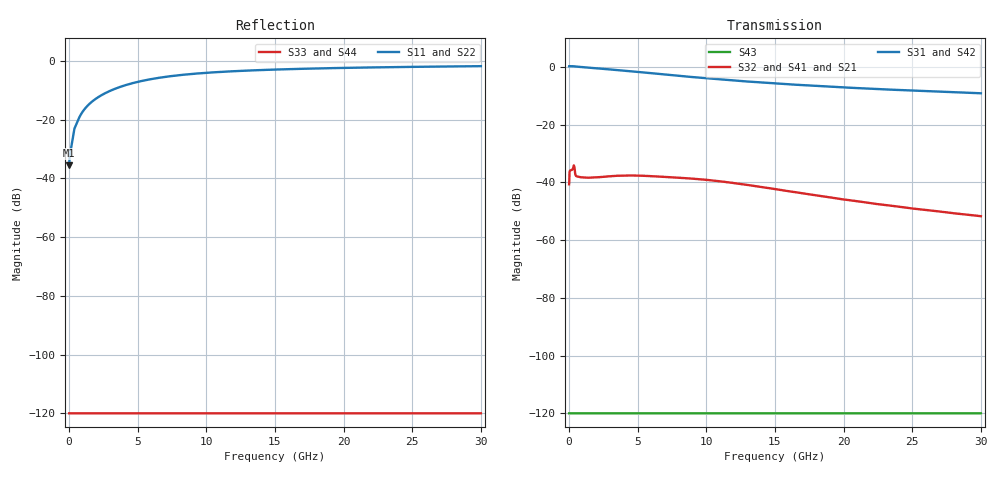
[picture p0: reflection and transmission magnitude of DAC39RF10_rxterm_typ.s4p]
! Copyright 2008, Texas Instruments Incorporated. All rights reserved.
! Generated by program util_convert_RxTerm_to_s4p on 03-29-2011 13:58:47
!  1 ----xxxxxxxxxxxxxxxxxx---- 3
!  xxxxxxxxxxxxxxxxxx
!  (Input) xxxxxxxxxxxxxxxxxx  (Output)
!  xxxxxxxxxxxxxxxxxx
!  2 ----xxxxxxxxxxxxxxxxxx---- 4
! FREQ  S11  S12  S13  S14
!  S21  S22  S23  S24
!  S31  S32  S33  S34
!  S41  S42  S43  S44
!  DB  ANG  DB  ANG  DB  ANG  DB  ANG
# HZ S DB R 50.00
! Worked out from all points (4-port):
!   3000 points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, 10 MHz to 30 GHz, reference 50 ohm
!   strongest paths, dB at 10 MHz, 7.51 GHz, 15.01 GHz, 22.51 GHz, 30 GHz:
!     S31: 0.1, -2.9, -5.8, -7.7, -9.2
!     S42: 0.2, -2.9, -5.8, -7.8, -9.2
!     S32: -40.7, -38.3, -42.4, -47.6, -51.7
!     S41: -40.7, -38.5, -42.4, -47.6, -51.7
!     S21: -40.7, -38.5, -42.4, -47.6, -51.7
!     S43: -120.0, -120.0, -120.0, -120.0, -120.0
!   lowest |S11| = -35.5 dB at 20 MHz (marker M1), VSWR 1.03, Z = 51.7 + j0.154 ohm
!   |S11| at or under -10 dB: start of sweep to 3.086 GHz
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1e7  -35.14 -9.5  -40.70 -7.4  -120.00 0.0  -120.00 0.0
     -40.69 -7.7  -35.04 -9.3  -120.00 0.0  -120.00 0.0
     0.15 -0.2  -40.70 -7.4  -120.00 0.0  -120.00 0.0
     -40.69 -7.7  0.15 -0.2  -120.00 0.0  -120.00 0.0
2e7  -35.53 5.1  -40.08 29.0  -120.00 0.0  -120.00 0.0
     -40.17 28.8  -35.40 5.0  -120.00 0.0  -120.00 0.0
     0.14 0.1  -40.08 29.0  -120.00 0.0  -120.00 0.0
     -40.17 28.8  0.15 0.1  -120.00 0.0  -120.00 0.0
5e8  -21.95 -86.1  -37.78 -19.3  -120.00 0.0  -120.00 0.0
     -37.74 -19.6  -21.88 -86.0  -120.00 0.0  -120.00 0.0
     0.07 -4.5  -37.78 -19.3  -120.00 0.0  -120.00 0.0
     -37.74 -19.6  0.08 -4.6  -120.00 0.0  -120.00 0.0
1.28e9  -15.61 -104.9  -38.41 -11.2  -120.00 0.0  -120.00 0.0
        -38.43 -11.6  -15.54 -105.1  -120.00 0.0  -120.00 0.0
        -0.26 -9.5  -38.41 -11.2  -120.00 0.0  -120.00 0.0
        -38.43 -11.6  -0.26 -9.6  -120.00 0.0  -120.00 0.0
5.1e9  -7.03 -127.4  -37.70 -32.9  -120.00 0.0  -120.00 0.0
       -37.83 -33.2  -6.99 -127.6  -120.00 0.0  -120.00 0.0
       -1.83 -25.9  -37.70 -32.9  -120.00 0.0  -120.00 0.0
       -37.83 -33.2  -1.84 -26.0  -120.00 0.0  -120.00 0.0
1.412e10  -3.08 -149.6  -41.72 -94.5  -120.00 0.0  -120.00 0.0
          -41.80 -93.8  -3.08 -149.8  -120.00 0.0  -120.00 0.0
          -5.50 -42.0  -41.72 -94.5  -120.00 0.0  -120.00 0.0
          -41.80 -93.8  -5.54 -41.9  -120.00 0.0  -120.00 0.0
3e10  -1.79 -161.3  -51.74 -137.4  -120.00 0.0  -120.00 0.0
      -51.70 -136.7  -1.80 -161.3  -120.00 0.0  -120.00 0.0
      -9.18 -48.8  -51.74 -137.4  -120.00 0.0  -120.00 0.0
      -51.70 -136.7  -9.19 -48.5  -120.00 0.0  -120.00 0.0
